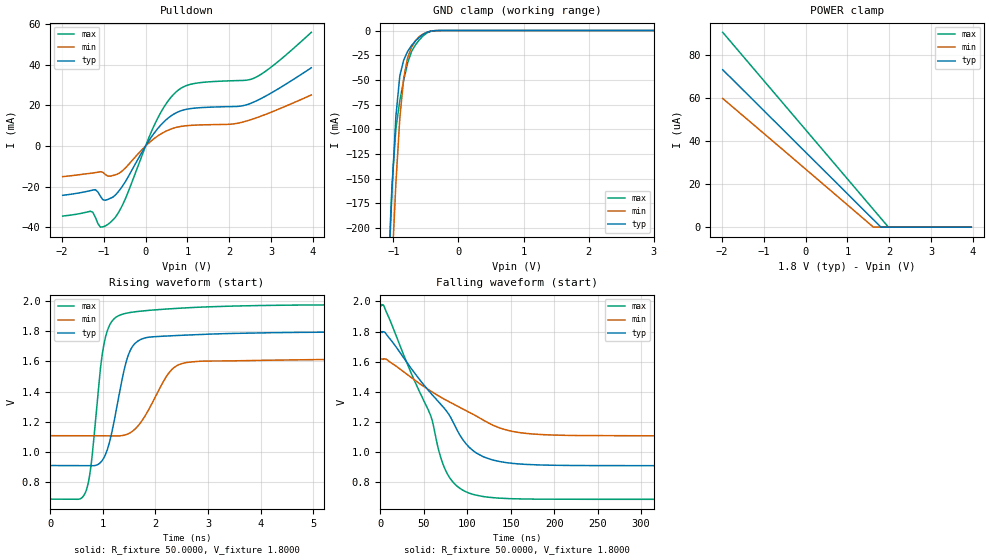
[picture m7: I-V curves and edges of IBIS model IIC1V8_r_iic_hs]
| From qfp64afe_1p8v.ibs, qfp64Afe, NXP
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[Model] IIC1V8_r_iic_hs
|   Model IIC1V8_r_iic_hs
| This model was characterised for following simulation conditions:
| External (pad) voltage:
|   - Typ: 1.8V,   - Min: 1.62V,   - Max: 1.98V
| Library cells for typ/min/max conditions are connected as defined below:
|  IO - External Pad
|  A - Core Input
|  EN - Output Buffer Enable
|  BOOST - vdde
|  ECS - gnd
|  EGP - gnd
|  ENZI - vdd
|  EPD - vdd
|  EPUN - gnd
|  ZI - NC
|  ZIF - NC
|  gnd - gnd
|  gnde - gnde
|  vdd - vdd
|  vdde - vdde
| All other pins connected to ground
Model_type I/O_open_drain
Polarity   Non-Inverting
Enable   Active-Low
Vinl =   0.5400V
Vinh =   1.2600V
Vmeas =  0.9000V
Cref =   0.0F
Rref =   1000.000
Vref =   1.8000V
C_comp   3.6138pF   3.4666pF   3.7547pF
|C_comp_pullup   0.9378pF   0.9163pF   0.9441pF
|C_comp_pulldown   2.3253pF   2.4781pF   2.1797pF
[Model Spec]
| variable   typ   min   max
Vinh   0.5400V   0.4860V   0.5940V
Vinl   1.2600V   1.1340V   1.3860V
Vmeas   0.9000V   0.8100V   0.9900V
Vref   1.8000V   1.6200V   1.9800V
Cref   0.0F   0.0F   0.0F
Rref   1.0000k   1.0000k   1.0000k
[Temperature Range]   25.0000   0.1250k   -40.0000
[Voltage Range]   1.8000V   1.6200V   1.9800V
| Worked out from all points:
|   slope of the pulldown table from 0 to 0.27 V, typ, clamps not added: 33.4 ohm
|   GND clamp passes 1 mA (typ) near -0.44 V on its own axis
|   rising waveform, R_fixture 50.0000, V_fixture 1.8000: 20-80 % time 320ps typ, 490ps min, 236ps max; typ from 0.91 V to 1.8 V
|   falling waveform, R_fixture 50.0000, V_fixture 1.8000: 20-80 % time 66.8ns typ, 88.5ns min, 48.9ns max; typ from 1.8 V to 0.91 V
[Pulldown]
|Voltage   I(typ)   I(min)   I(max)
-1.98V    -24.22mA   -15.04mA   -34.42mA
-1.32V    -21.94mA   -13.4mA    -32.06mA
-1.2V     -21.45mA   -13.05mA   -35.06mA
-1.08V    -24.63mA   -12.6mA    -39.9mA
-900mV    -26.23mA   -14.78mA   -38.53mA
-540mV    -19.33mA   -11.9mA    -28.53mA
300mV     8.856mA    5.096mA    14.12mA
720mV     16.26mA    9.117mA    26.48mA
1.14V     18.6mA     10.26mA    30.69mA
2.1V      19.45mA    10.89mA    32.16mA
2.58V     21.61mA    13.43mA    33.34mA
3.96V     38.53mA    25.17mA    55.97mA
[GND_clamp]
|Voltage   I(typ)   I(min)   I(max)
-1.98V    -2.104A    -2.075A    -2.136A
-1.08V    -259.3mA   -333mA     -246.9mA
-1.02V    -161.8mA   -238.7mA   -157.1mA
-960mV    -86.75mA   -154.7mA   -99.47mA
-900mV    -45.96mA   -88.82mA   -71.06mA
-840mV    -29.91mA   -48mA      -50.26mA
-780mV    -21.16mA   -27.65mA   -32.99mA
-720mV    -15.17mA   -16.88mA   -21.27mA
-660mV    -10.57mA   -10.24mA   -14.57mA
-540mV    -3.796mA   -3.405mA   -5.301mA
-300mV    -21.69uA   -40.85uA   -23.15uA
3.96V     0A         0A         0A
[POWER_clamp]
|Voltage   I(typ)   I(min)   I(max)
-1.98V    73.06uA    59.72uA    90.42uA
1.62V     3.484uA    0A         8.225uA
1.8V      0A         0A         4.113uA
1.98V     0A         0A         0A
3.96V     0A         0A         0A
[Ramp]
| variable   typ   min   max
dV/dt_r  0.5328/0.3203n   0.3064/0.4904n   0.7742/0.2363n
dV/dt_f  0.5327/66.8193n   0.3063/88.5501n   0.7742/48.8599n
R_load = 50.0000
[Rising Waveform]
R_fixture= 50.0000
V_fixture= 1.8000
V_fixture_min= 1.6200
V_fixture_max= 1.9800
|time   V(typ)   V(min)   V(max)
0s        910.3mV    1.108V     687.5mV
683.5ps   909.6mV    1.108V     745.3mV
781.7ps   908.4mV    1.108V     930.9mV
1.005ns   953mV      1.108V     1.685V
1.257ns   1.283V     1.106V     1.895V
1.482ns   1.642V     1.121V     1.923V
1.767ns   1.752V     1.22V      1.935V
2.501ns   1.774V     1.586V     1.954V
5.893ns   1.796V     1.615V     1.976V
1us       1.798V     1.619V     1.978V
[Falling Waveform]
R_fixture= 50.0000
V_fixture= 1.8000
V_fixture_min= 1.6200
V_fixture_max= 1.9800
|time   V(typ)   V(min)   V(max)
0s        1.798V     1.619V     1.978V
4.165ns   1.798V     1.62V      1.971V
57.81ns   1.394V     1.407V     1.245V
67.61ns   1.331V     1.372V     1.004V
75.49ns   1.278V     1.346V     875.1mV
91.61ns   1.113V     1.297V     760.2mV
112.4ns   988.6mV    1.234V     712.3mV
146.4ns   929.9mV    1.145V     692.5mV
203.2ns   913.1mV    1.113V     688.1mV
1us       910.4mV    1.108V     687.5mV
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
